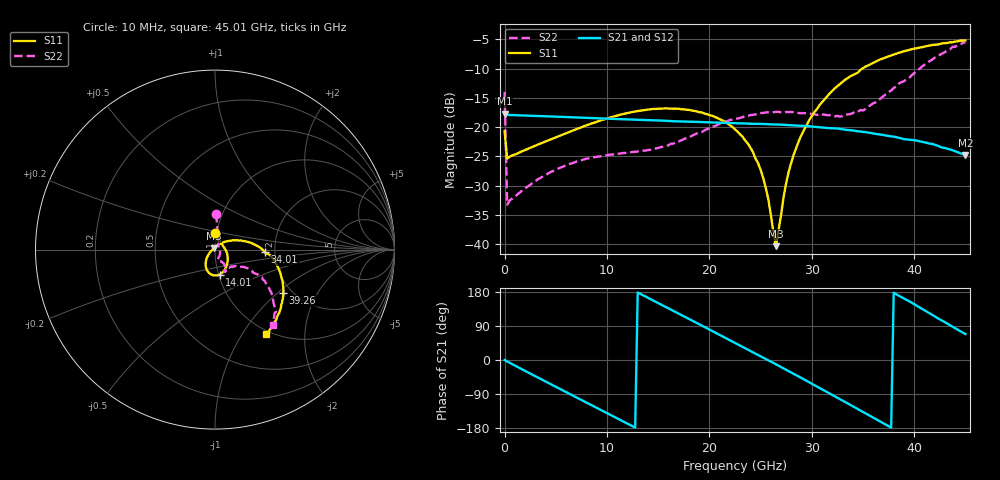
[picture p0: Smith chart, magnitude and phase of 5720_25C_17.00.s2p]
! Device:  ADRF5720
! Description: 0.5dB LSB GaAs MMIC 6-bit Digital Attenuator
! Frequency:  0.000009 -  40 GHz
! Ports:
!	RF1	= Port 1
!	RF2	= Port 2
! Vdd:  3.3 Volt
! Vss:  -3.3 Volt
! Control:  0/3.3 Volt
! State:  17.00 dB attenuation
! Data:  The device was measured using G-S-G Probes on a matrix board.
!  Data was collected using an calibrated 4 port network analyzer.
!  The reference plane for this measurement is at the launchers.
! Note:  Analog Devices supplies this data as a sample of measured data
!  for this product.  Your particular data for this product may vary.
!  Data was taken at 25 degrees C.
!  Analog Devices reserves the right to change this data at anytime.
# GHZ S DB R 45.0
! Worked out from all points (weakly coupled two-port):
!   181 points, 10 MHz to 45.01 GHz, reference 45 ohm
!   highest |S21| = -17.72 dB at 10 MHz (marker M1); lowest = -24.8 dB at 45.01 GHz (marker M2)
!   lowest |S11| = -40.4 dB at 26.51 GHz (marker M3), VSWR 1.02, Z = 44.4 + j0.616 ohm
!   |S11| at or under -10 dB: start of sweep to 34.94 GHz
!   |S22| runs from -33.3 to -5.5 dB; largest |S21 - S12| = 0.00016
!   S11 on the Smith chart (normalised r, x): 10 MHz: 0.98, +0.18; 14.01 GHz: 1.01, -0.29; 34.01 GHz: 1.77, -0.06; 39.26 GHz: 1.80, -1.09; 45.01 GHz: 0.95, -1.28
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0.01  -20.67 90.5  -17.72 -0.2  -17.72 -0.2  -13.98 87.9
0.26  -25.39 8.9  -17.91 -3.9  -17.92 -3.9  -33.26 21.5
3.26  -22.99 -17.9  -18.11 -46.4  -18.10 -46.4  -28.92 -38.6
7.76  -19.85 -47.3  -18.40 -109.0  -18.40 -109.0  -25.52 -70.4
14.01  -17.00 -79.6  -18.81 164.2  -18.81 164.2  -23.92 -71.3
15.26  -16.83 -85.6  -18.88 146.7  -18.88 146.7  -23.43 -67.6
19.26  -17.50 -105.0  -19.14 90.9  -19.14 91.0  -20.85 -58.5
22.76  -20.77 -125.0  -19.35 41.9  -19.35 41.9  -18.54 -59.9
24.01  -23.50 -134.4  -19.43 24.3  -19.43 24.3  -17.95 -61.8
25.01  -27.29 -143.6  -19.45 10.1  -19.45 10.1  -17.60 -63.4
25.76  -32.27 -159.7  -19.51 -0.7  -19.51 -0.7  -17.46 -64.5
26.51  -40.35 133.8  -19.56 -11.4  -19.56 -11.4  -17.39 -65.9
27.26  -31.89 64.3  -19.61 -22.4  -19.61 -22.4  -17.54 -65.9
27.76  -27.56 49.8  -19.66 -29.6  -19.67 -29.5  -17.43 -66.3
28.76  -22.27 36.1  -19.75 -44.0  -19.75 -44.0  -17.61 -67.1
30.26  -17.46 23.1  -19.93 -66.2  -19.94 -66.2  -17.78 -65.0
32.01  -13.79 10.5  -20.20 -91.9  -20.20 -91.8  -18.05 -59.7
34.01  -11.12 -3.0  -20.57 -122.1  -20.58 -122.0  -17.62 -45.8
37.76  -7.74 -24.3  -21.57 -178.5  -21.57 -178.4  -13.76 -29.9
39.26  -6.94 -32.3  -22.11 158.9  -22.12 159.0  -11.80 -30.7
42.01  -5.93 -45.8  -23.01 115.1  -23.01 115.1  -8.13 -37.1
45.01  -5.19 -59.0  -24.75 68.4  -24.75 68.5  -5.48 -52.3
